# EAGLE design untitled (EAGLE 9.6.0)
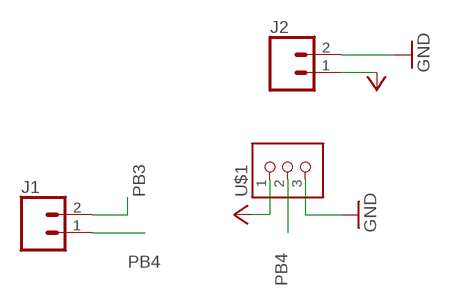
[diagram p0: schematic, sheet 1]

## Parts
J1  CONN_02  [1X02]
J2  CONN_02  [1X02]
U$1  CONN_03_TERM'-FABLAB'  [ED555DS-3DS]

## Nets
GND: J2.2 U$1.3
PB3: J1.2
PB4: J1.1 U$1.2
VCC: J2.1 U$1.1

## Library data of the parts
J1 J2 = SparkFun-Connectors:CONN_02: Multi connection point. Often used as Generic Header-pin footprint for 0.1 inch spaced/style header connections
U$1 = fab:CONN_03_TERM: 3.5mm terminal block, 3 positions ED555-3DS as found in the fablab inventory. Made by Zaerc.

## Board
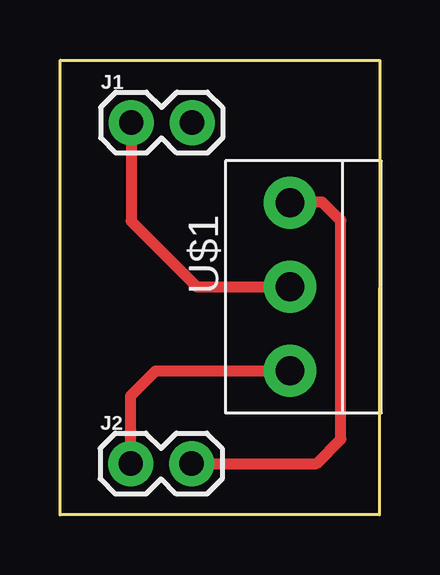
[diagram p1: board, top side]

Size 13.33 x 18.95 mm. Coordinates in mm from the lower left corner, seen from the top.
Outline: 0.01,18.95 13.33,18.93 13.31,0 0,0 0.01,18.95
Copper layers (1*16): Top 0.035mm / dielectric 1.5mm / Bottom 0.035mm
Design rules "default *": minimum track width 18mil, minimum drill 0.35mm, track to track 16mil, track to pad 16mil, pad to pad 16mil, via to via 6mil, smd to smd 16mil, copper to edge 40mil, drill to drill 6mil, minimum pad ring 10mil, minimum via ring 8mil, stop-mask expansion 4mil, vias tented up to drill 0mil, thermal gap 10mil

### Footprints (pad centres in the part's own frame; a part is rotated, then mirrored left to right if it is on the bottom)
1X02 = drill 1.016 pad 1.88: 1 0,0; 2 2.54,0
ED555DS-3DS = drill 1.2 pad 2.184: 1 -3.5,0; 2 0,0; 3 3.5,0

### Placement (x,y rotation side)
J1  2.97,16.34 0 top
J2  2.95,2.13 0 top
U$1  9.59,9.5 90 top

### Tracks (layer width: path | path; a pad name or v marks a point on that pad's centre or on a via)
GND
  Top 0.457: J2.2 10.69,2.13 11.7,3.15 11.7,12.25 10.92,13.03 9.62,13.03 U$1.3
PB4
  Top 0.457: J1.1 2.97,12.24 5.71,9.5 U$1.2
VCC
  Top 0.457: J2.1 2.95,4.96 3.99,6 U$1.1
